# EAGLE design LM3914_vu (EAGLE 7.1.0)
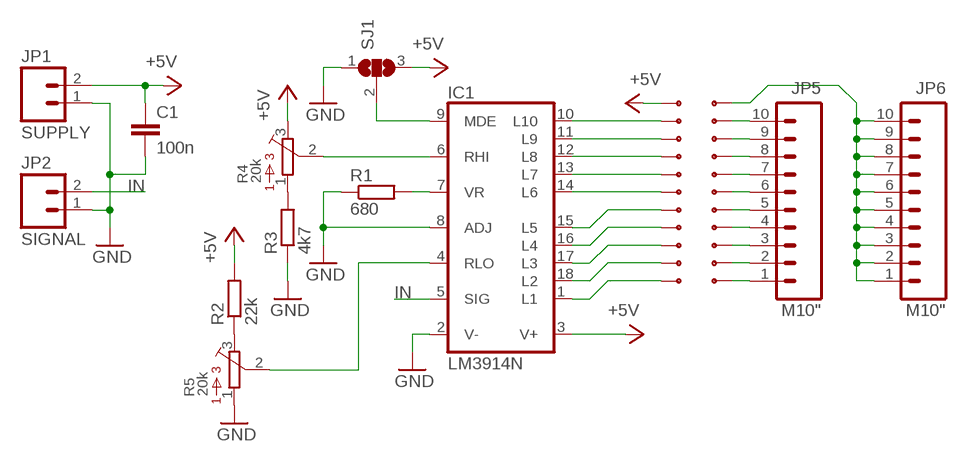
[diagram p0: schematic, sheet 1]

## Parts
C1  100n  C-EU025-030X050  [C025-030X050]
IC1  LM3914N  [DIL18]
JP1  SUPPLY  M02PTH  [1X02]
JP2  SIGNAL  M02PTH  [1X02]
JP5  M10"  [1X10]
JP6  M10"  [1X10]
P1  SMD-PAD  [SMD-PAD]
P2  SMD-PAD  [SMD-PAD]
P3  SMD-PAD  [SMD-PAD]
P4  SMD-PAD  [SMD-PAD]
P5  SMD-PAD  [SMD-PAD]
P6  SMD-PAD  [SMD-PAD]
P7  SMD-PAD  [SMD-PAD]
P8  SMD-PAD  [SMD-PAD]
P9  SMD-PAD  [SMD-PAD]
P10  SMD-PAD  [SMD-PAD]
P11  SMD-PAD  [SMD-PAD]
P12  SMD-PAD  [SMD-PAD]
P13  SMD-PAD  [SMD-PAD]
P14  SMD-PAD  [SMD-PAD]
P15  SMD-PAD  [SMD-PAD]
P16  SMD-PAD  [SMD-PAD]
P17  SMD-PAD  [SMD-PAD]
P18  SMD-PAD  [SMD-PAD]
P19  SMD-PAD  [SMD-PAD]
P20  SMD-PAD  [SMD-PAD]
P21  SMD-PAD  [SMD-PAD]
P22  SMD-PAD  [SMD-PAD]
R1  680  R-EU_0204/2V  [0204V]
R2  22k  R-EU_0204/2V  [0204V]
R3  4k7  R-EU_0204/2V  [0204V]
R4  20k  3386-F  [3386F]
R5  20k  3386-F  [3386F]
SJ1  JUMPER  [JUMPER]

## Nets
+5V: C1.1 IC1.3(V+) JP1.2 P3.P$1 R2.2 R4.3 SJ1.3
COM: JP6.1 JP6.2 JP6.3 JP6.4 JP6.5 JP6.6 JP6.7 JP6.8 JP6.9 JP6.10 P1.P$1
GND: C1.2 IC1.2(V-) IC1.8(ADJ) JP1.1 JP2.1 R1.1 R3.1 R5.1 SJ1.1
IN: IC1.5(SIG) JP2.2
N$1: IC1.14(L6) P8.P$1
N$2: IC1.18(L2) P12.P$1
N$3: IC1.13(L7) P7.P$1
N$4: IC1.16(L4) P10.P$1
N$5: IC1.15(L5) P9.P$1
N$6: IC1.12(L8) P6.P$1
N$7: IC1.17(L3) P11.P$1
N$8: IC1.11(L9) P5.P$1
N$9: IC1.1(L1) P13.P$1
N$10: IC1.10(L10) P4.P$1
N$11: IC1.7(VR) R1.2
N$12: R3.2 R4.1
N$13: IC1.9(MDE) SJ1.2
N$14: IC1.6(RHI) R4.2
N$15: IC1.4(RLO) R5.2
N$16: R2.1 R5.3
N$17: JP5.1 P22.P$1
N$18: JP5.2 P21.P$1
N$19: JP5.3 P20.P$1
N$20: JP5.4 P19.P$1
N$21: JP5.5 P18.P$1
N$22: JP5.6 P17.P$1
N$23: JP5.7 P16.P$1
N$24: JP5.8 P15.P$1
N$25: JP5.9 P14.P$1
N$26: JP5.10 P2.P$1

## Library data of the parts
C1 = rcl:C-EU: CAPACITOR, European symbol
IC1 = linear:LM3914N: LED DRIVER senses analog voltage levels and drives 10 LEDs
JP1 JP2 = SparkFun-Connectors:M02: Standard 2-pin 0.1" header. Use with
JP5 JP6 = SparkFun-Connectors:M10: Header 10 Standard 10-pin 0.1" header. Use with straight break away headers (SKU : PRT-00116), right angle break away headers (PRT-00553), swiss pins (PRT-00743), machine pins (PRT-00117), and female headers (PRT-00115).
P1-P22 = 1Axel:SMD-PAD
R1-R3 = rcl:R-EU_: RESISTOR, European symbol
R4 R5 = Bourns:3386-: 3386 Series 3/8" Square Trimmer
SJ1 = Axel:JUMPER

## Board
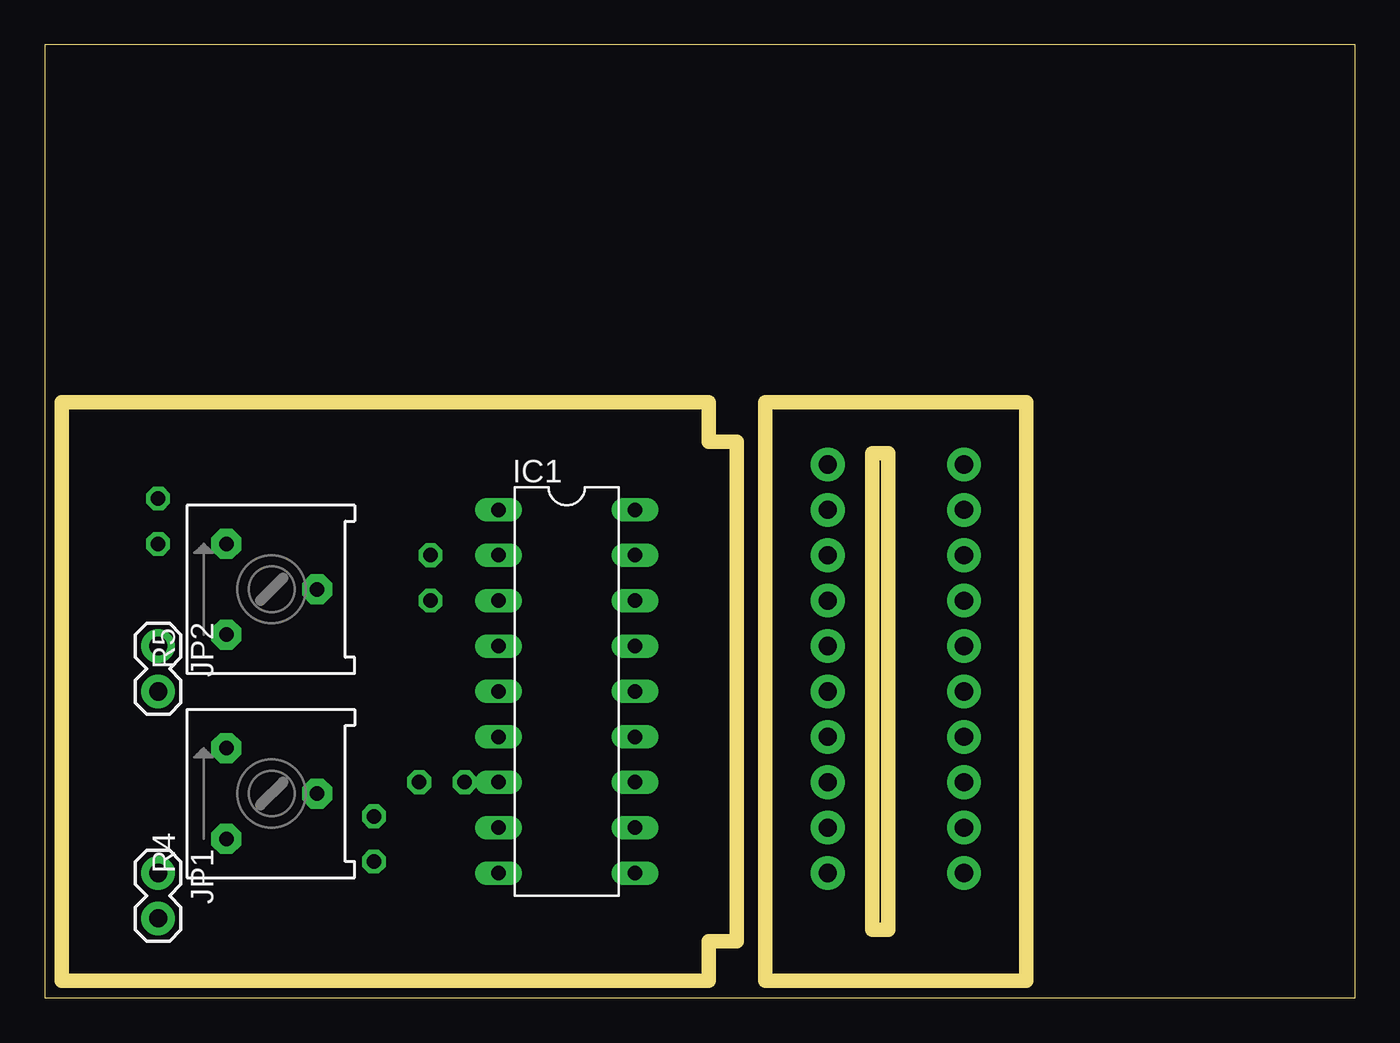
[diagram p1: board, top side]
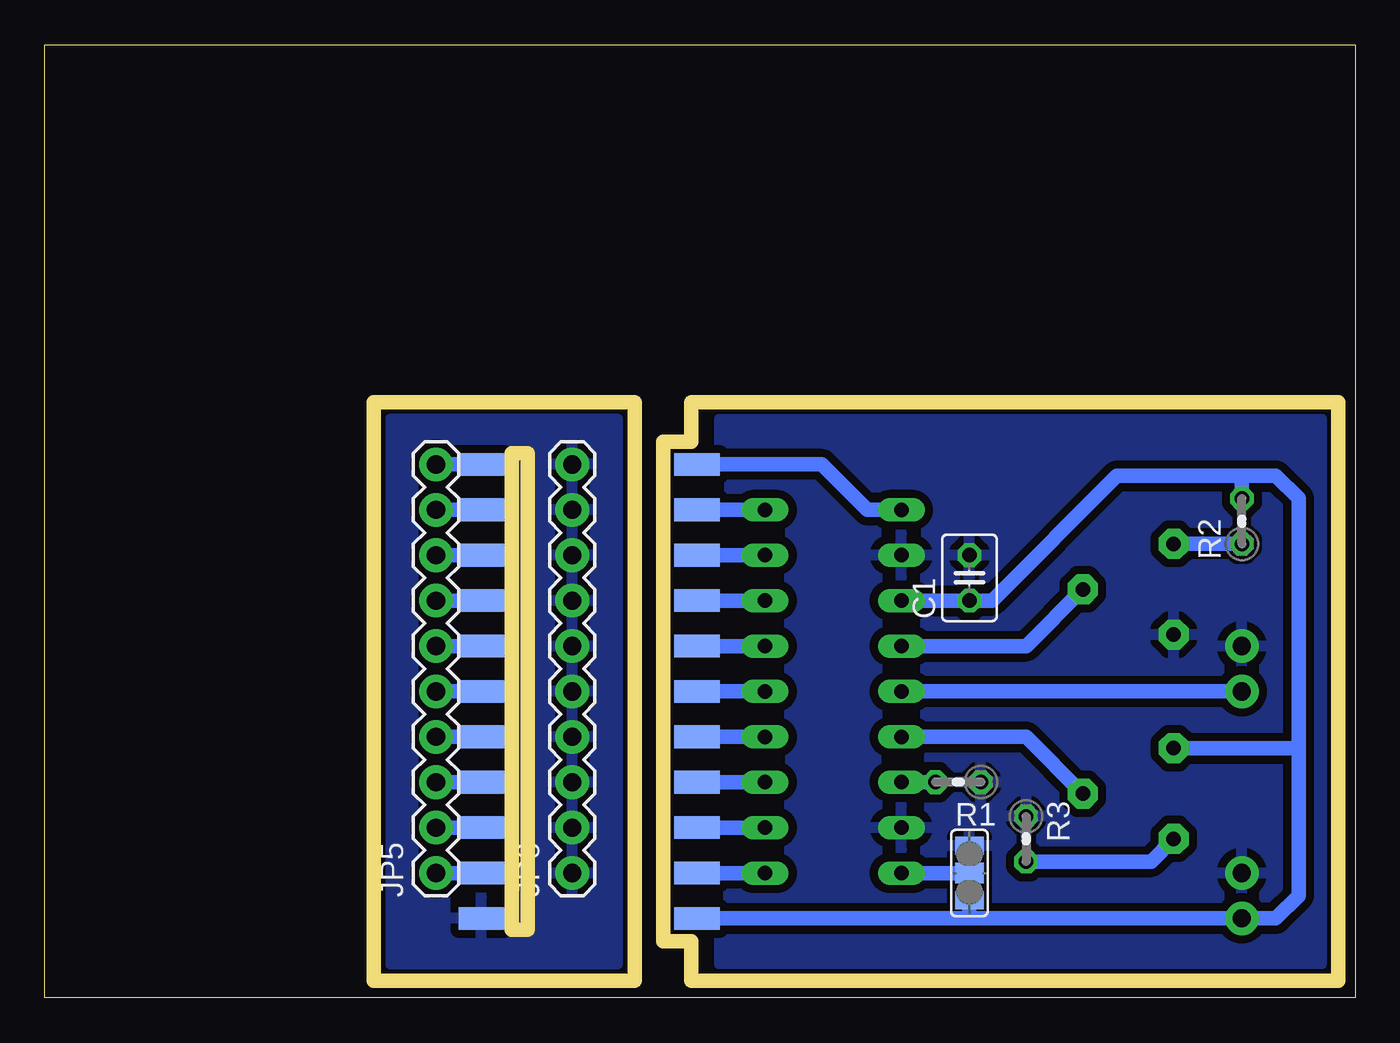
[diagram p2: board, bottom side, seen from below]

Size 73.33 x 53.33 mm. Coordinates in mm from the lower left corner, seen from the top.
Outline: 0,0 73.33,0 73.33,53.33 0,53.33 0,0
Copper layers (1*16): Top 0.035mm / dielectric 1.5mm / Bottom 0.035mm
Design rules "default *": minimum track width 10mil, minimum drill 24mil, track to track 0.36mm, track to pad 0.36mm, pad to pad 0.36mm, via to via 0.36mm, smd to smd 0.36mm, copper to edge 40mil, drill to drill 8mil, minimum pad ring 10mil, minimum via ring 8mil, stop-mask expansion 4mil, vias tented up to drill 0mil, thermal gap 0.46mm
Milling: 16 lines

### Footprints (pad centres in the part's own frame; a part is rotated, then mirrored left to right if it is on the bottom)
C025-030X050 = drill 0.813 octagon: 1 -1.27,0; 2 1.27,0
DIL18 = drill 0.813 long: 1 -10.16,-3.81; 2 -7.62,-3.81; 3 -5.08,-3.81; 4 -2.54,-3.81; 5 0,-3.81; 6 2.54,-3.81; 7 5.08,-3.81; 8 7.62,-3.81; 9 10.16,-3.81; 10 10.16,3.81; 11 7.62,3.81; 12 5.08,3.81; 13 2.54,3.81; 14 0,3.81; 15 -2.54,3.81; 16 -5.08,3.81; 17 -7.62,3.81; 18 -10.16,3.81
1X02 = drill 1.016 pad 1.88: 1 0,0; 2 2.54,0
1X10 = drill 1.016 pad 1.88: 1 0,0; 2 2.54,0; 3 5.08,0; 4 7.62,0; 5 10.16,0; 6 12.7,0; 7 15.24,0; 8 17.78,0; 9 20.32,0; 10 22.86,0
SMD-PAD = smd 1.27 x 2.54: P$1 0,0
0204V = drill 0.813 octagon: 1 -1.27,0; 2 1.27,0
3386F = drill 0.813 pad 1.676 octagon: 1 -2.54,2.54; 2 0,-2.54; 3 2.54,2.54
JUMPER = smd 1 x 1.6: 1 -1.524,0; 3 1.524,0 | smd 1.168 x 1.6: 2 0,0

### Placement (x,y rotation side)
C1  21.59,23.5 90 bottom
IC1  29.21,17.14 270 top
JP1  6.35,6.99 270 top
JP2  6.35,19.68 270 top
JP5  51.44,6.99 90 bottom
JP6  43.81,6.99 90 bottom
P1  48.9,4.45 270 bottom
P2  48.9,29.84 270 bottom
P3  36.83,4.45 270 bottom
P4  36.83,6.99 270 bottom
P5  36.83,9.53 270 bottom
P6  36.83,12.06 270 bottom
P7  36.83,14.61 270 bottom
P8  36.83,17.14 270 bottom
P9  36.83,19.68 270 bottom
P10  36.83,22.23 90 bottom
P11  36.83,24.77 90 bottom
P12  36.83,27.3 90 bottom
P13  36.83,29.84 90 bottom
P14  48.9,27.3 270 bottom
P15  48.9,24.77 270 bottom
P16  48.9,22.23 270 bottom
P17  48.9,19.68 270 bottom
P18  48.9,17.14 270 bottom
P19  48.9,14.61 270 bottom
P20  48.9,12.06 270 bottom
P21  48.9,9.53 270 bottom
P22  48.9,6.99 270 bottom
R1  22.23,12.06 180 bottom
R2  6.35,26.67 90 bottom
R3  18.41,8.89 270 bottom
R4  12.7,11.43 90 top
R5  12.7,22.86 90 top
SJ1  21.59,6.99 270 bottom

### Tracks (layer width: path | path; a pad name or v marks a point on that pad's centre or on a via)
+5V
  Bottom 0.813: IC1.3 C1.1 20.32,22.23 13.34,29.21 6.35,29.21 | 3.17,13.97 3.17,5.71 4.45,4.45 JP1.2 21.59,4.45 | 3.17,13.97 3.17,27.94 4.45,29.21 6.35,29.21 | R4.3 3.17,13.97 | P3.P$1 21.59,4.45 | R2.2 6.35,29.21 | SJ1.3 21.59,4.45
COM
  pour Bottom (isolate 0.46): 53.98,1.91 41.27,1.91 41.27,32.38 53.98,32.38
GND
  pour Bottom (isolate 0.46): 1.91,1.91 35.56,1.91 35.56,32.38 1.91,32.38
IN
  Bottom 0.813: IC1.5 JP2.2
N$1
  Bottom 0.813: IC1.14 P8.P$1
N$2
  Bottom 0.813: IC1.18 P12.P$1
N$3
  Bottom 0.813: IC1.13 P7.P$1
N$4
  Bottom 0.813: IC1.16 P10.P$1
N$5
  Bottom 0.813: IC1.15 P9.P$1
N$6
  Bottom 0.813: IC1.12 P6.P$1
N$7
  Bottom 0.813: IC1.17 P11.P$1
N$8
  Bottom 0.813: IC1.11 P5.P$1
N$9
  Bottom 0.813: IC1.1 27.3,27.3 29.84,29.84 P13.P$1
N$10
  Bottom 0.813: IC1.10 P4.P$1
N$11
  Bottom 0.813: R1.2 IC1.7
N$12
  Bottom 0.813: R3.2 11.43,7.62 R4.1
N$13
  Bottom 0.813: SJ1.2 IC1.9
N$14
  Bottom 0.813: IC1.6 18.41,14.61 R4.2
N$15
  Bottom 0.813: IC1.4 18.41,19.68 R5.2
N$16
  Bottom 0.813: R2.1 R5.3
N$17
  Bottom 0.8: P22.P$1 JP5.1
N$18
  Bottom 0.8: P21.P$1 JP5.2
N$19
  Bottom 0.8: P20.P$1 JP5.3
N$20
  Bottom 0.8: P19.P$1 JP5.4
N$21
  Bottom 0.8: P18.P$1 JP5.5
N$22
  Bottom 0.8: P17.P$1 JP5.6
N$23
  Bottom 0.8: P16.P$1 JP5.7
N$24
  Bottom 0.8: P15.P$1 JP5.8
N$25
  Bottom 0.8: P14.P$1 JP5.9
N$26
  Bottom 0.8: JP5.10 P2.P$1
